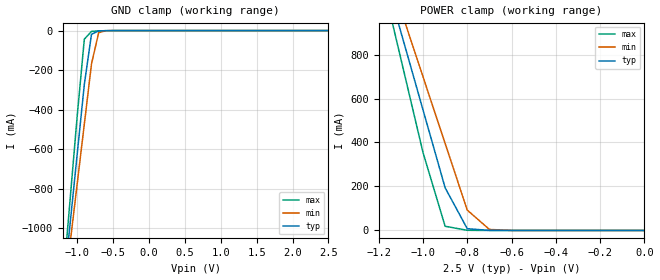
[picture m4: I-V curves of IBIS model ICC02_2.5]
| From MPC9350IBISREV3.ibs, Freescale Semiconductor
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|   ICC02_2.5: LVCMOS INPUT MODEL WITH A 25K PULLUP RESISTOR
[Model]   ICC02_2.5
Model_type  Input
Vinh   =  1.7
Vinl   =  0.7
C_comp   4pF   4pF   4pF
[Temperature Range] 55   110   0
[Voltage Range]   2.5   2.25   2.75
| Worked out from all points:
|   GND clamp passes 1 mA (typ) near -0.64 V on its own axis
|   POWER clamp passes 1 mA (typ) near -0.71 V on its own axis
[GND Clamp]
-2.5V     -5.968A    -5.351A    -6.849A
-1.2V     -1.34A     -1.387A    -1.291A
-1.1V     -983.9mA   -1.082A    -863.3mA
-1V       -628.2mA   -777.7mA   -436mA
-900mV    -272.6mA   -473.3mA   -43.61mA
-800mV    -18.37mA   -169.1mA   -4.071mA
-700mV    -1.803mA   -10.53mA   -1.748mA
-600mV    -469.6uA   -844.1uA   -549.6uA
2.5V      142.9pA    38.25nA    18.64pA
[POWER Clamp]
-2.5V     5.872A     5.257A     6.751A
-1.2V     1.258A     1.306A     1.207A
-1.1V     903mA      1.003A     780.7mA
-1V       548.5mA    699.1mA    354.8mA
-900mV    194.1mA    395.6mA    19.11mA
-800mV    7.956mA    92.59mA    801.4uA
-700mV    419.3uA    4.687mA    153.6uA
-600mV    61.5uA     290.9uA    36.86uA
0V        142.9pA    662pA      21.65pA
